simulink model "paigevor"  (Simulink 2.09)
settings: Solver=ode45  StartTime=0  StopTime=5.0  MaxStep=.01  RelTol=1e-3  AbsTol=1e-3

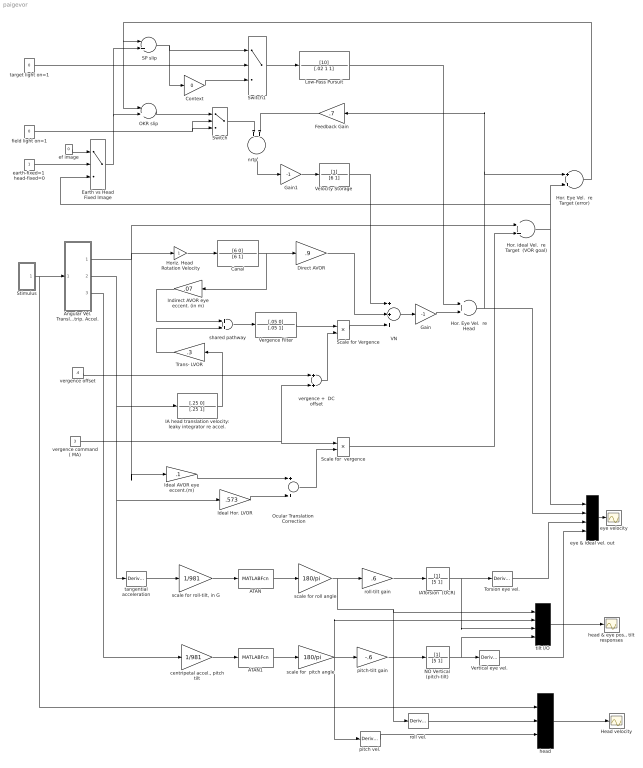
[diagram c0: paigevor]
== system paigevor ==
  " SP slip" : Sum  Inputs=-+
  ATAN : MATLABFcn  MATLABFcn=atan  OutputWidth=-1
  ATAN1 : MATLABFcn  MATLABFcn=atan  OutputWidth=-1
  Angular Vel. Translation Vel. Centrip. Accel. : Subsystem
  Canal : TransferFcn  Numerator=[6 0]  Denominator=[6 1]
  Context : Gain  Gain=0
  Direct AVOR : Gain  Gain=.9
  Earth vs Head Fixed Image : Switch  Threshold=.5
  Feedback Gain : Gain  Orientation=left  Gain=.7
  Gain : Gain  Gain=-1
  Gain1 : Gain  Gain=-1
  Head velocity : Scope
  Hor. Eye Vel.  re Head : Sum  Inputs=++
  Hor. Eye Vel.  re Target (error) : Sum  Inputs=++
  Hor. ideal Vel.  re Target  (VOR goal) : Sum  Inputs=++
  Horiz. Head  Rotation Velocity : Gain  Gain=1
  IA head translation velocity: leaky integrator re accel. : TransferFcn  Numerator=[.25 0]  Denominator=[.25 1]
  IATorsion  (OCR) : TransferFcn  Numerator=[1]  Denominator=[5 1]
  Ideal AVOR eye eccent.(m) : Gain  Gain=.1
  Ideal Hor. LVOR : Gain  Gain=.573
  Indirect AVOR eye eccent. (in m) : Gain  Orientation=left  Gain=.07
  Low-Pass Pursuit : TransferFcn  Numerator=[10]  Denominator=[.02 1 1]
  NO Vertical (pitch-tilt) : TransferFcn  Numerator=[1]  Denominator=[5 1]
  OKR slip : Sum  Inputs=-+
  Ocular Translation  Correction : Sum  Inputs=++
  Scale for Vergence : Product  Inputs=2
  "Scale for  vergence " : Product  Inputs=2
  Stimulus : Subsystem
  Switch : Switch  Threshold=.5
  Switch1 : Switch  Threshold=.5
  Torsion eye vel. : Derivative
  Trans- LVOR : Gain  Orientation=left  Gain=.3
  VN : Sum  Inputs=+++
  "Velocity Storage " : TransferFcn  Numerator=[1]  Denominator=[6 1]
  Vergence Filter : TransferFcn  Numerator=[.05 0]  Denominator=[.05 1]
  Vertical eye vel. : Derivative
  "centripetal accel., pitch tilt" : Gain  Gain=1/981
  earth-fixed=1  head-fixed=0 : Constant  Value=1
  ef image : Constant  Value=0
  eye & ideal vel. out : Mux  Inputs=4
  eye velocity : Scope
  field light on=1 : Constant  Value=0
  head : Mux  Inputs=3
  "head & eye pos., tilt responses" : Scope
  nrtp : Sum  Orientation=down  Inputs=++
  pitch vel. : Derivative
  pitch-tilt gain : Gain  Gain=-.6
  roll vel. : Derivative
  roll-tilt gain : Gain  Gain=.6
  scale for roll angle : Gain  Gain=180/pi
  scale for  pitch angle : Gain  Gain=180/pi
  "scale for roll-tilt, in G" : Gain  Gain=1/981
  shared pathway : Sum  Inputs=++
  tangential acceleration : Derivative
  target light on=1 : Constant  Value=0
  tilt I/O : Mux  Inputs=4
  vergence command ( MA) : Constant  Value=3
  vergence +  DC offset : Sum  Inputs=++
  vergence offset : Constant  Value=.4
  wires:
  head/1 -> Head velocity/1
  pitch vel./1 -> head/3
  roll vel./1 -> head/2
  vergence command ( MA)/1 -> vergence +  DC offset/2, "Scale for  vergence "/1
  vergence offset/1 -> vergence +  DC offset/1
  vergence +  DC offset/1 -> Scale for Vergence/2
  IA head translation velocity: leaky integrator re accel./1 -> Trans- LVOR/1
  eye & ideal vel. out/1 -> eye velocity/1
  NO Vertical (pitch-tilt)/1 -> tilt I/O/4, Vertical eye vel./1
  IATorsion  (OCR)/1 -> tilt I/O/3, Torsion eye vel./1
  roll-tilt gain/1 -> IATorsion  (OCR)/1
  scale for roll angle/1 -> roll vel./1, tilt I/O/1, roll-tilt gain/1
  tilt I/O/1 -> "head & eye pos., tilt responses"/1
  scale for  pitch angle/1 -> tilt I/O/2, pitch vel./1, pitch-tilt gain/1
  " SP slip"/1 -> Context/1, Switch1/1
  ef image/1 -> Earth vs Head Fixed Image/1
  Context/1 -> Switch1/3
  Switch1/1 -> Low-Pass Pursuit/1
  target light on=1/1 -> Switch1/2
  field light on=1/1 -> Switch/3, Switch/2
  Stimulus/1(out_1) -> head/1, Angular Vel. Translation Vel. Centrip. Accel./1(Inport)
  Canal/1 -> Indirect AVOR eye eccent. (in m)/1, Direct AVOR/1
  shared pathway/1 -> Vergence Filter/1
  Direct AVOR/1 -> VN/2
  Scale for Vergence/1 -> VN/3
  tangential acceleration/1 -> "scale for roll-tilt, in G"/1
  pitch-tilt gain/1 -> NO Vertical (pitch-tilt)/1
  "centripetal accel., pitch tilt"/1 -> ATAN1/1
  ATAN1/1 -> scale for  pitch angle/1
  earth-fixed=1  head-fixed=0/1 -> Earth vs Head Fixed Image/2
  Angular Vel. Translation Vel. Centrip. Accel./3(centrip. linear  accel. stimulus) -> "centripetal accel., pitch tilt"/1
  ATAN/1 -> scale for roll angle/1
  "scale for roll-tilt, in G"/1 -> ATAN/1
  Low-Pass Pursuit/1 -> Hor. Eye Vel.  re Head/1
  "Scale for  vergence "/1 -> Hor. ideal Vel.  re Target  (VOR goal)/2
  Ocular Translation  Correction/1 -> "Scale for  vergence "/2
  Ideal AVOR eye eccent.(m)/1 -> Ocular Translation  Correction/1
  Ideal Hor. LVOR/1 -> Ocular Translation  Correction/2
  Gain/1 -> Hor. Eye Vel.  re Head/2
  "Velocity Storage "/1 -> VN/1
  Switch/1 -> nrtp/1
  OKR slip/1 -> Switch/1
  Feedback Gain/1 -> nrtp/2
  nrtp/1 -> Gain1/1
  Gain1/1 -> "Velocity Storage "/1
  VN/1 -> Gain/1
  Vergence Filter/1 -> Scale for Vergence/1
  Trans- LVOR/1 -> shared pathway/2
  Indirect AVOR eye eccent. (in m)/1 -> shared pathway/1
  Horiz. Head  Rotation Velocity/1 -> Canal/1
  Vertical eye vel./1 -> eye & ideal vel. out/4
  Torsion eye vel./1 -> eye & ideal vel. out/3
  Hor. Eye Vel.  re Head/1 -> Hor. Eye Vel.  re Target (error)/1, Feedback Gain/1, eye & ideal vel. out/2
  Angular Vel. Translation Vel. Centrip. Accel./2(tangential linear velocity stimulus) -> tangential acceleration/1, Ideal Hor. LVOR/1, IA head translation velocity: leaky integrator re accel./1
  Angular Vel. Translation Vel. Centrip. Accel./1(hor. rotation velocity  stimulus) -> Ideal AVOR eye eccent.(m)/1, Hor. ideal Vel.  re Target  (VOR goal)/1, Horiz. Head  Rotation Velocity/1
  Earth vs Head Fixed Image/1 -> " SP slip"/2, OKR slip/2
  Hor. Eye Vel.  re Target (error)/1 -> OKR slip/1, " SP slip"/1
  Hor. ideal Vel.  re Target  (VOR goal)/1 -> Hor. Eye Vel.  re Target (error)/2, Earth vs Head Fixed Image/3, eye & ideal vel. out/1

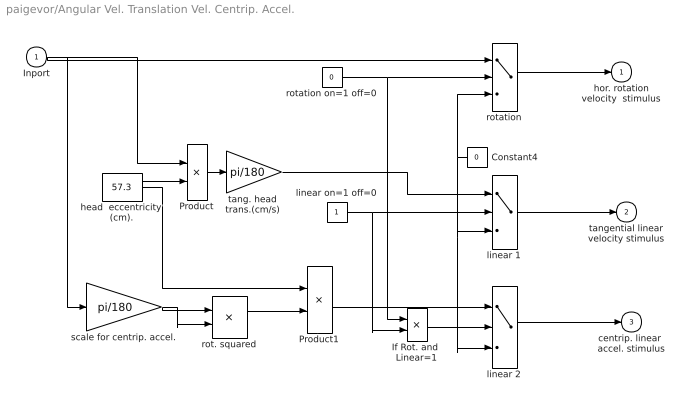
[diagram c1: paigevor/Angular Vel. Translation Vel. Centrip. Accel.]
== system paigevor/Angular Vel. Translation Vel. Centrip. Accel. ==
  Inport : Inport  Port=1  PortWidth=-1  SampleTime=-1
  Constant4 : Constant  Orientation=left  Value=0
  If Rot. and  Linear=1 : Product  Inputs=2
  Product : Product  Inputs=2
  Product1 : Product  Inputs=2
  head  eccentricity (cm). : Constant  Value=57.3
  linear 1 : Switch  Threshold=.5
  linear 2 : Switch  Threshold=.5
  linear on=1 off=0 : Constant  Value=1
  rot. squared : Product  Inputs=2
  rotation : Switch  Threshold=.5
  rotation on=1 off=0 : Constant  Value=0
  scale for centrip. accel. : Gain  Gain=pi/180
  "tang. head  trans.(cm/s) " : Gain  Gain=pi/180
  hor. rotation velocity  stimulus : Outport  Port=1  InitialOutput=0
  tangential linear velocity stimulus : Outport  Port=2  InitialOutput=0
  centrip. linear  accel. stimulus : Outport  Port=3  InitialOutput=0
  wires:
  scale for centrip. accel./1 -> rot. squared/2, rot. squared/1
  linear 1/1 -> tangential linear velocity stimulus/1
  linear 2/1 -> centrip. linear  accel. stimulus/1
  Product1/1 -> linear 2/1
  head  eccentricity (cm)./1 -> Product1/1, Product/2
  rot. squared/1 -> Product1/2
  Inport/1 -> scale for centrip. accel./1, Product/1, rotation/1
  "tang. head  trans.(cm/s) "/1 -> linear 1/1
  Product/1 -> "tang. head  trans.(cm/s) "/1
  rotation/1 -> hor. rotation velocity  stimulus/1
  Constant4/1 -> rotation/3, linear 2/3, linear 1/3
  If Rot. and  Linear=1/1 -> linear 2/2
  rotation on=1 off=0/1 -> rotation/2, If Rot. and  Linear=1/1
  linear on=1 off=0/1 -> linear 1/2, If Rot. and  Linear=1/2

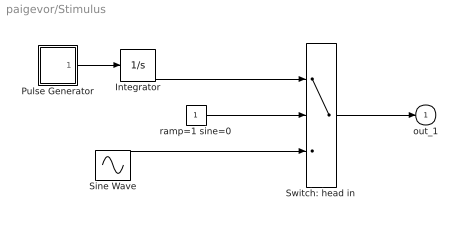
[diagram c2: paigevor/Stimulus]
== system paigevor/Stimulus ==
  Integrator : Integrator  ExternalReset=none  InitialConditionSource=internal  InitialCondition=0  LimitOutput=off  UpperSaturationLimit=inf  LowerSaturationLimit=-inf  ShowSaturationPort=off  ShowStatePort=off  AbsoluteTolerance=auto
  Pulse Generator : Subsystem  mask(Pulse Generator){}
      mask help: Pulse Generator.
      mask init:
      | Ts=@1; du=@2; ht=@3; stt=@4; ini=ones(length(ht),1); st1=rem(stt,Ts); st2=rem(stt+du,Ts);if(Ts<=1.2*du),ini=zeros(length(ht),1);end;
  Sine Wave : Sin  Amplitude=20  Frequency=4*pi*2  Phase=0  SampleTime=-1
  Switch: head in : Switch  Threshold=.5
  ramp=1 sine=0 : Constant  Value=1
  out_1 : Outport  Port=1  InitialOutput=0
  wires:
  Switch: head in/1 -> out_1/1
  Integrator/1 -> Switch: head in/1
  Sine Wave/1 -> Switch: head in/3
  ramp=1 sine=0/1 -> Switch: head in/2
  Pulse Generator/1(out_1) -> Integrator/1

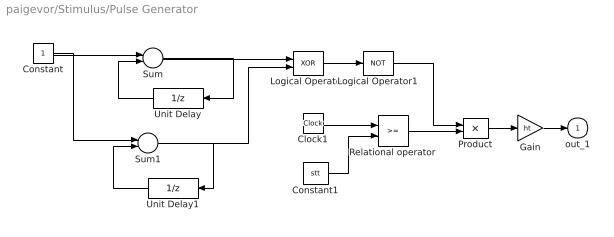
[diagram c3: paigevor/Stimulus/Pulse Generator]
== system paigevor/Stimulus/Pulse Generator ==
  Clock1 : Clock
  Constant : Constant  Value=1
  Constant1 : Constant  Value=stt
  Gain : Gain  Gain=ht
  Logical Operator : Logic  Operator=XOR  Inputs=2
  Logical Operator1 : Logic  Operator=NOT  Inputs=1
  Product : Product  Inputs=2
  Relational operator : RelationalOperator  Operator=>=
  Sum : Sum  Inputs=+-
  Sum1 : Sum  Inputs=+-
  Unit Delay : UnitDelay  Orientation=left  X0=0  SampleTime=[Ts,st1]
  Unit Delay1 : UnitDelay  Orientation=left  X0=ini  SampleTime=[Ts,st2]
  out_1 : Outport  Port=1  InitialOutput=0
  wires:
  Sum1/1 -> Logical Operator/2, Unit Delay1/1
  Sum/1 -> Logical Operator/1, Unit Delay/1
  Constant/1 -> Sum1/1, Sum/1
  Unit Delay1/1 -> Sum1/2
  Unit Delay/1 -> Sum/2
  Clock1/1 -> Relational operator/1
  Relational operator/1 -> Product/2
  Product/1 -> Gain/1
  Gain/1 -> out_1/1
  Constant1/1 -> Relational operator/2
  Logical Operator/1 -> Logical Operator1/1
  Logical Operator1/1 -> Product/1
